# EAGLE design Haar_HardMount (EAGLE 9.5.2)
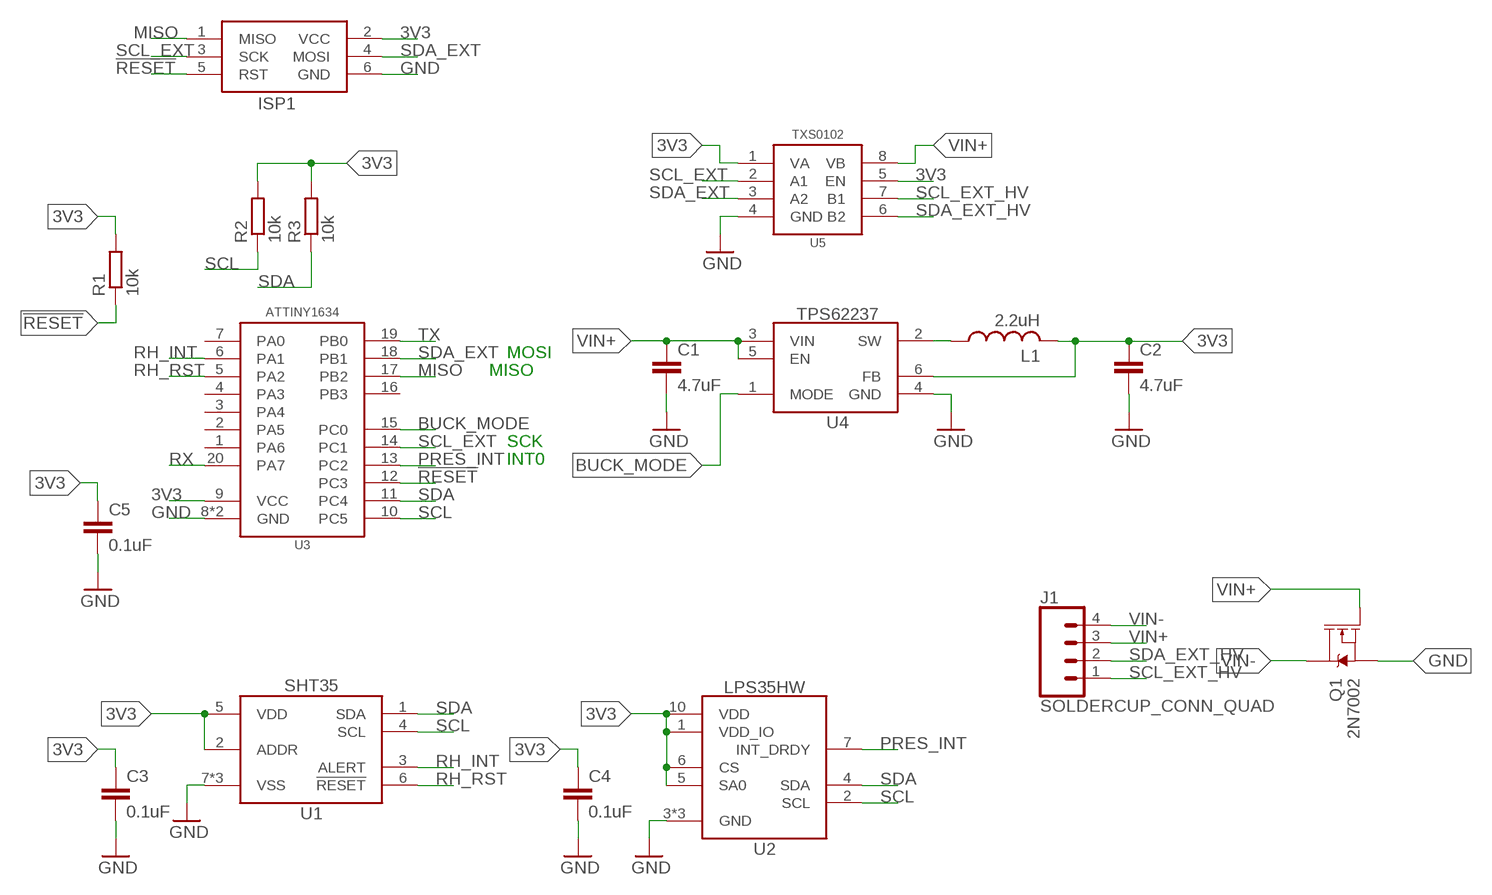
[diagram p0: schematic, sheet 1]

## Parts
C1  4.7uF  C-EUC0402  [C0402]
C2  4.7uF  C-EUC0402  [C0402]
C3  0.1uF  C-EU0.1UFC0402  [C0402]
C4  0.1uF  C-EU0.1UFC0402  [C0402]
C5  0.1uF  C-EU0.1UFC0402  [C0402]
ISP1  AVRISP1.27MM  [2X3_1.27]
J1  SOLDERCUP_CONN_QUAD  [SOLDERCUP_CONN_QUAD]
L1  2.2uH  INDUCTOR0805  [0805]
Q1  2N7002  MOSFET-NCH-2N7002PW  [SOT323]
R1  10k  R-EU_10KR0402  [R0402]
R2  10k  R-EU_10KR0402  [R0402]
R3  10k  R-EU_10KR0402  [R0402]
U1  SHT35DFN  [DFN_8_2.5X2.5]
U2  LPS35HW  [CCLGA10L]
U3  ATTINY1634QFN  [QFN20]
U4  TPS62237DRY  [DRY0006A]
U5  TXS0102DQM  [DQM_R-PX2SON-N8]

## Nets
3V3: C2.1 C3.1 C4.1 C5.1 ISP1.2(VCC) L1.2 R1.2 R2.2 R3.2 U1.2(ADDR) U1.5(VDD) U2.1(VDD_IO) U2.5(SA0) U2.6(CS) U2.10(VDD) U3.9(VCC) U4.6(FB) U5.1(VA) U5.5(EN)
!RESET: ISP1.5(RST) R1.1 U3.12(PC3)
BUCK_MODE: U3.15(PC0) U4.1(MODE)
GND: C1.2 C2.2 C3.2 C4.2 C5.2 ISP1.6(GND) Q1.2(S) U1.7(VSS) U1.8(VSS) U1.EP(VSS) U2.3(GND) U2.8(GND) U2.9(GND) U3.8(GND) U3.EP(GND) U4.4(GND) U5.4(GND)
MISO: ISP1.1(MISO) U3.17(PB2)
N$1: L1.1 U4.2(SW)
PRES_INT: U2.7(INT_DRDY) U3.13(PC2)
RH_INT: U1.3(ALERT) U3.6(PA1)
RH_RST: U1.6(!RESET) U3.5(PA2)
RX: U3.20(PA7)
SCL: R2.1 U1.4(SCL) U2.2(SCL) U3.10(PC5)
SCL_EXT: ISP1.3(SCK) U3.14(PC1) U5.2(A1)
SCL_EXT_HV: J1.1 U5.7(B1)
SDA: R3.1 U1.1(SDA) U2.4(SDA) U3.11(PC4)
SDA_EXT: ISP1.4(MOSI) U3.18(PB1) U5.3(A2)
SDA_EXT_HV: J1.2 U5.6(B2)
TX: U3.19(PB0)
VIN+: C1.1 J1.3 Q1.1(G) U4.3(VIN) U4.5(EN) U5.8(VB)
VIN-: J1.4 Q1.3(D)
Unconnected: U3.1(PA6) U3.2(PA5) U3.3(PA4) U3.4(PA3) U3.7(PA0) U3.16(PB3)

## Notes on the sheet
- MOSI
- MISO
- SCK
- INT0

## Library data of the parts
C1 C2 = bschulz_passives:C-EU: CAPACITOR, European symbol; DIGIKEY: 490-14306-1-ND; MF: Murata; MPN: GRM155R61A475MEAAD
C3-C5 = bschulz_passives:C-EU: CAPACITOR, European symbol; DIGIKEY: 490-4759-1-ND; MF: Murata; MPN: GCM155R71C104KA55D
ISP1 = bschulz:AVRISP: AVR ISP HEADER Standard 6 pin header for AVR programming
J1 = bschulz:SOLDERCUP_CONN_QUAD
L1 = bschulz:INDUCTOR: Genaric inductor; DIGIKEY: 732-2953-1-ND; MF: Wurth; MPN: 74479775222
Q1 = bschulz:MOSFET-NCH: N-channel MOSFETs Voltage controlled devices that allow control of high current outputs. SparkFun Products: SparkFun OpenScale SparkFun Digital Sandbox SparkFun Monster Moto Shield SparkFun MOSFET Power Controller; DIGIKEY: 2N7002W-FDICT-ND; MF: Diodes Incorporated; MPN: 2N7002W-7-F; PROD_ID: TRANS-11151
R1-R3 = bschulz_passives:R-EU_: RESISTOR, European symbol; DIGIKEY: 311-10.0KHRCT-ND; MF: Yageo; MPN: RC0603FR-0710KL; VALUE_PART: 10k
U1 = bschulz:SHT3*: SHT3x - Digital Humidity and Temperature Sensor Characteristics (for SHT35): Vcc: 2.15V ~ 5.5V Humidity Resolution: 0.01% RH Humidity Accuracy: &plusmn;1.5% RH Temperature Resolution: 0.01°C Temperature Accuracy: 0.1°C Operating Temperature: -40°C to 125°C Digikey: 1649-1065-1-ND (SHT30)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; DIGIKEY: 1649-1067-1-ND; DISP: SHT35; MF: Sensirion; MPN: SHT35-DIS-F2.5KS
U2 = bschulz:LPS3*HW: LPS3xHW - Digital Water Resistant Pressure Sensor Characteristics: Vcc: 1.7V ~ 3.6V Pressure Range: 260 ~ 1260 mBar Pressure Resolution: 0.24 &mu;Bar Pressure Accuracy: relative &plusmn;0.1 mBar, abs &plusmn; 1 mBar Temperature Resolution: 0.01°C Temperature Accuracy: 1.5°C Operating Temperature: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; DIGIKEY: 497-16706-1-ND; DISP: LPS35HW; MF: ST; MPN: LPS35HWTR
U3 = bschulz:ATTINY1634: ATtiny1634 8 bit AVR Microcontroller Features: Vcc: 1.8 ~ 5.5V Clock: Up to 16MHz, Internal 8MHz FRC, 32kHz RC Flash Memory: 16K SRAM: 1K EEPROM: 256B ADC: 10b, 12 port USART: Yes, x2 SPI: Yes I2C: Yes, slave only Notes: 2 analog comp. Digikey: ATTINY1634R-MURCT-ND (QFN) ATTINY1634R-SU-ND (SOIC); DIGIKEY: ATTINY1634-MURCT-ND; MF: Atmel; MPN: ATTINY1634-MUR
U4 = bschulz:TPS6223*: TPS6223xx - Ultra Small Step Down Converter (Buck) Characteristics: Vin: 2.05V ~ 6V Vout: 1V ~ 3.3V (fixed increments) IQ: 22&mu;A Output Current: 500 mA Operating Temperature: -40°C to 85°C Digikey: TPS62237 (3.3V Fixed); DIGIKEY: 296-39454-1-ND; DISP: TPS62237; MF: TI; MPN: TPS62237DRYR
U5 = bschulz:TXS0102: TXS0102 - 2 Channel Bidirectional Voltage Level Translator Characteristics: Vcc: 1.65 ~ 3.6V (Port A), 2.3 ~ 5.5V (Port B) IQ: 14.4&mu;A Output Current: 50mA Output Type: Open Drain/Push-Pull Operating Temperature: -40°C to 85°C Digikey: 296-28368-1-ND (DQE) 296-28435-1-ND (DQM) 296-21931-1-ND (DCU); DIGIKEY: 296-28435-1-ND; MF: TI; MPN: TXS0102DQMR

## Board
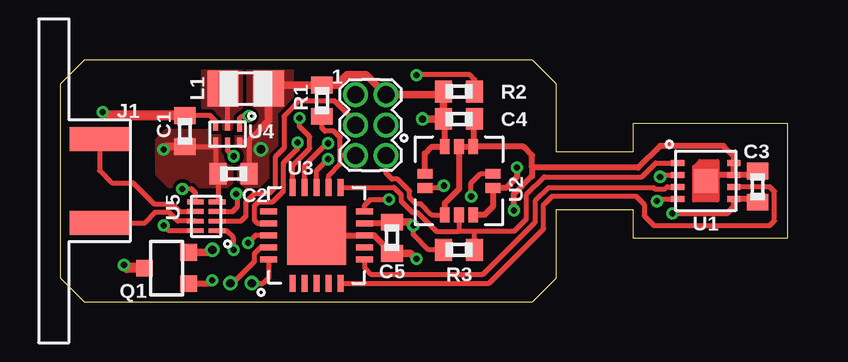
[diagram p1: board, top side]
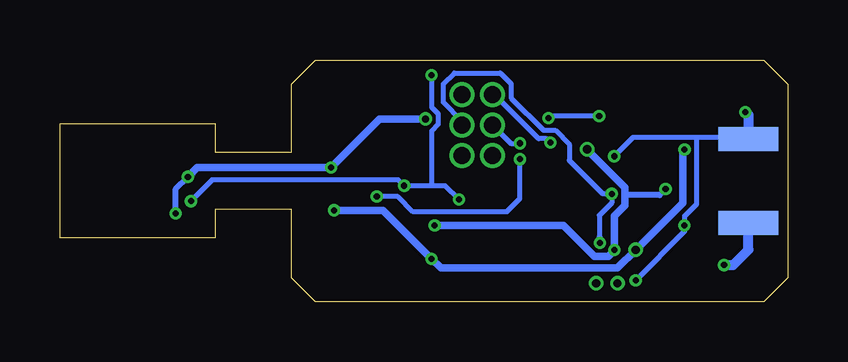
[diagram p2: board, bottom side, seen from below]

Size 30.35 x 10.08 mm. Coordinates in mm from the lower left corner, seen from the top.
Outline: 20.7,6.23 20.7,9.08 19.7,10.08 1,10.08 0,9.08 0,1 1,0 19.7,0 20.7,1 20.7,3.85 23.88,3.85 23.88,2.66 30.35,2.66 30.35,7.42 23.88,7.42 23.88,6.23 20.7,6.23
Copper layers (1*16): Top 0.035559375mm / dielectric 1.6mm / Bottom 0.035559375mm
Design rules "oshpark-2layer": minimum track width 6mil, minimum drill 10mil, track to track 6mil, track to pad 6mil, pad to pad 6mil, via to via 6mil, smd to smd 6mil, copper to edge 15mil, drill to drill 6mil, minimum pad ring 5mil, minimum via ring 5mil, stop-mask expansion 2.5mil, vias tented up to drill 0mil, thermal gap 10mil

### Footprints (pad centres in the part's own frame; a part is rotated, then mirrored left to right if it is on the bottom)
C0402 = smd 0.7 x 0.9: 1 -0.65,0; 2 0.65,0
2X3_1.27 = drill 0.7 pad 1.05: 1 -1.27,-0.635; 2 -1.27,0.635; 3 0,-0.635; 4 0,0.635; 5 1.27,-0.635; 6 1.27,0.635
SOLDERCUP_CONN_QUAD = smd 1 x 2.5: 1 1.75,1.27; 2 -1.75,1.27 | smd 1 x 2.5 bottom: 3 -1.75,1.27; 4 1.75,1.27
0805 = smd 1.3 x 1.5: 1 -0.95,0; 2 0.95,0
SOT323 = smd 0.7 x 0.7: 1 -0.65,-0.925; 2 0.65,-0.925; 3 0,0.925
R0402 = smd 0.7 x 0.9: 1 -0.65,0; 2 0.65,0
DFN_8_2.5X2.5 = smd 0.55 x 0.25: 1 -1.175,0.75; 2 -1.175,0.25; 3 -1.175,-0.25; 4 -1.175,-0.75; 5 1.175,-0.75; 6 1.175,-0.25; 7 1.175,0.25; 8 1.175,0.75 | smd 1 x 1: EP 0,0
CCLGA10L = smd 0.63 x 0.4: 1 -1.42,0.3; 2 -1.42,-0.3; 6 1.42,-0.3; 7 1.42,0.3 | smd 0.4 x 0.63: 3 -0.6,-1.42; 4 0,-1.42; 5 0.6,-1.42; 8 0.6,1.42; 9 0,1.42; 10 -0.6,1.42
QFN20 = smd 0.7 x 0.25: 1 -2.032,0.968; 2 -2.032,0.468; 3 -2.032,-0.032; 4 -2.032,-0.532; 5 -2.032,-1.032; 11 1.968,-1.032; 12 1.968,-0.532; 13 1.968,-0.032; 14 1.968,0.468; 15 1.968,0.968 | smd 0.25 x 0.7: 6 -1.032,-2.032; 7 -0.532,-2.032; 8 -0.032,-2.032; 9 0.468,-2.032; 10 0.968,-2.032; 16 0.968,1.968; 17 0.468,1.968; 18 -0.032,1.968; 19 -0.532,1.968; 20 -1.032,1.968 | smd 2.45 x 2.45: EP -0.032,-0.032
DRY0006A = smd 0.35 x 0.2: 1 -0.275,0.5 | smd 0.3 x 0.2: 2 -0.3,0; 3 -0.3,-0.5; 4 0.3,-0.5; 5 0.3,0; 6 0.3,0.5
DQM_R-PX2SON-N8 = smd 0.2 x 0.7: 1 -0.6,-0.45; 2 -0.2,-0.45; 3 0.2,-0.45; 4 0.6,-0.45; 5 0.6,0.45; 6 0.2,0.45; 7 -0.2,0.45; 8 -0.6,0.45

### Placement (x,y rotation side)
C1  5.21,7.11 270 top
C2  7.24,5.33 180 top
C3  29.08,4.8 90 top
C4  16.64,7.62 0 top
C5  13.84,2.67 270 top
ISP1  12.95,7.37 270 top
J1  0.38,5.04 270 top
L1  7.75,8.89 0 top
Q1  4.45,1.4 90 top
R1  10.92,8.38 90 top
R2  16.64,8.76 180 top
R3  16.64,2.16 180 top
U1  26.92,5.04 0 top
U2  16.64,5.04 0 top
U3  10.67,2.79 90 top
U4  6.99,6.99 270 top
U5  6.1,3.56 90 top

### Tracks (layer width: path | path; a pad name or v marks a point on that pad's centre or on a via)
3V3  (via drill 0.25, 0.3, 0.35)
  Top 0.2: U5.5 5.65,4.54 5.48,4.7 v5.1,4.7 | 6.76,2.96 U5.1 6.95,2.96 7.24,2.67 v7.24,2.16 | 8.38,7.24 7.89,6.75 7.89,6.68 | 7.89,6.68 C2.1 | U4.6 7.89,6.68 | v25.02,5.21 25.1,5.29 U1.2 | R3.2 15.37,2.16 14.73,2.79 v14.73,3.17
  Top 0.254: U2.1 15.22,6.19 15.49,6.46 U2.10 16.04,7.57 C4.1 | 28.93,4.25 C3.1 28.94,4.29 U1.5 28.1,3.97 27.81,3.68 v25.53,3.68 | v19.05,5.59 19.05,5.21 18.59,4.74 U2.6 18.06,3.97 17.71,3.62 U2.5 | C5.1 13.79,3.26 U3.9
  Top 0.305: 8.38,7.24 8.7,7.55 L1.2 8.84,9.03 R1.2 11.54,9.03 11.97,9.47 12.76,9.47 ISP1.2 15.86,8.64 R2.2 C4.1 v15.11,7.62 | v14.73,3.17 14.59,3.32 C5.1
  Bottom 0.254: v25.53,3.68 25.53,4.7 v25.02,5.21 | v19.05,5.59 | v5.1,4.7 5.36,4.45 6.79,4.45
  Bottom 0.305: v19.05,5.59 24.64,5.59 v25.02,5.21 | v14.73,3.17 9.35,3.17 8.07,1.89 7.48,1.89 7.24,2.13 v7.24,2.16 7.24,3.56 6.79,4.01 6.79,4.45 6.79,4.76 v8.38,6.35 | v19.05,5.59 17.02,7.62 v15.11,7.62
  pour Top (rank 2, no thermals): 7.87,9.65 7.87,7.24 7.75,7.11 7.37,7.11 7.37,5.21 7.75,4.83 8.26,4.83 9.65,6.22 9.65,9.78 9.53,9.91 8.13,9.91
!RESET
  Top 0.2: ISP1.5 11.68,6.1 | 11.68,6.1 11.68,6.84 11.41,7.11 11.05,7.11 10.92,7.24 R1.1 | 11.68,6.1 11.68,6.09 11.68,5.73 11.2,5.25 U3.12
BUCK_MODE  (via drill 0.25)
  Top 0.2: U4.1 7.49,7.64 7.58,7.74 v7.87,7.74 | v9.98,7.65 9.98,7.31 10.41,6.88 10.41,6.39 9.7,5.68 U3.15
  Bottom 0.2: v7.87,7.74 9.9,7.74 v9.98,7.65
GND  (via drill 0.25, 0.35)
  Top 0.2: ISP1.6 13.59,5.37 13.84,5.11 14.07,5.11 14.58,4.61 14.58,4.34 14.84,4.07 15.05,4.07 15.5,3.62 U2.3 | U4.4 6.49,6.48 | 6.49,6.48 6.49,5.44 C2.2 6.59,4.2 U5.4 | C1.2 6.47,6.46 6.49,6.48
  Top 0.254: U2.8 U2.9 16.64,4.7 16.04,4.1 U2.3 | C4.2 17.24,7.57 U2.8 | U1.7 U1.8 28.1,6.06 27.66,6.5 25.01,6.5 24.1,5.59 19.68,5.59 | 28.94,5.25 C3.2 28.98,5.29 U1.7 | C5.2 13.1,2.76 U3.8 U3.EP | v18.92,3.81 v18.93,3.81 18.93,4.47 19.68,5.24 19.68,5.59 | 19.68,5.59 19.68,6.1 19.32,6.46 U2.8 | 27.17,5.25 U1.EP 27.17,5.29 U1.7
  Top 0.305: v4.32,6.35 4.43,6.46 C1.2 | v14.86,1.78 14.62,2.02 C5.2 | v6.35,2.16 6.24,2.05 Q1.2
  Bottom 0.305: v4.32,6.35 4.39,6.27 4.39,4.12 v6.35,2.16 7.11,1.4 14.48,1.4 v14.86,1.78 16.89,3.81 v18.92,3.81
  pour Top (no thermals): 4.45,7.11 6.6,7.11 6.73,6.99 6.73,6.22 7.11,5.84 7.11,4.95 6.99,4.83 4.57,4.83 4.06,5.33 4.06,6.73
MISO  (via drill 0.25)
  Top 0.2: v9.91,6.64 9.91,6.39 9.32,5.8 9.32,4.62 8.84,4.14 8.24,4.14 8.1,3.99 8.1,3.4 8.24,3.26 U3.17
  Bottom 0.2: ISP1.1 12.24,8.64 10.39,6.79 10.06,6.79 v9.91,6.64
N$1
  Top 0.2: U4.2 6.99,8.7 L1.1
  pour Top (rank 3, no thermals): 6.73,7.37 6.86,7.24 7.11,7.24 7.24,7.37 7.24,7.75 7.62,8.13 7.62,9.65 7.49,9.78 6.1,9.78 5.97,9.65 5.97,8.13 6.22,7.87 6.6,7.87 6.73,7.75
PRES_INT  (via drill 0.25)
  Top 0.2: v17.14,4.38 17.14,4.95 17.53,5.34 U2.7 | U3.13 10.7,5.47 v11.18,5.94
  Bottom 0.2: v17.14,4.38 16.27,4.38 15.63,3.75 11.73,3.75 11.18,4.3 v11.18,5.94
RH_INT
  Top 0.2: U3.6 12.7,1.4 12.95,1.14 17.64,1.14 19.81,3.31 19.81,4.19 20.37,4.75 24.76,4.75 24.81,4.7 25.23,4.7 25.32,4.79 U1.3
RH_RST
  Top 0.2: U3.5 17.89,0.76 20.16,3.04 20.16,4.04 20.53,4.4 24.01,4.4 24.36,4.05 24.36,3.58 24.77,3.17 29.59,3.17 29.79,3.37 29.79,4.6 29.59,4.79 U1.6
RX  (via drill 0.35)
  Top 0.2: U3.20 8.7,1 8.46,0.76 v8,0.76
SCL  (via drill 0.25)
  Top 0.2: U3.10 12.7,4.02 12.94,4.26 v13.72,4.26 | v24.89,4.19 24.99,4.29 U1.4 | v16,4.83 15.91,4.74 U2.2 | v14.86,9.45 14.88,9.46 17.09,9.46 17.29,9.27 R2.1
  Bottom 0.2: v13.72,4.26 14.29,4.83 14.86,4.83 | 14.86,4.83 v16,4.83 16.26,5.09 24,5.09 v24.89,4.19 | v14.86,9.45 14.86,8.12 14.58,7.84 14.58,7.4 14.86,7.12 14.86,4.83
SCL_EXT  (via drill 0.25)
  Top 0.2: ISP1.3 12.32,7.49 11.43,8.38 10,8.38 9.34,7.72 9.34,6.4 8.97,6.04 8.97,4.77 8.69,4.49 8.1,4.49 7.75,4.14 7.75,3.56 7.54,3.36 U5.2 | U3.14 10.2,5.68 11.12,6.6 v11.18,6.6
  Bottom 0.2: ISP1.3 11.56,6.6 v11.18,6.6
SCL_EXT_HV
  Top 0.2: U5.7 4.91,3.36 4.54,3.73 3.98,3.73 3.55,3.29 J1.1
SDA
  Top 0.2: U2.4 16.64,2.93 | 17.29,2.93 18.93,2.93 19.43,3.43 19.43,4.45 20.19,5.21 24.26,5.21 24.84,5.79 U1.1 | 17.29,2.93 16.64,2.93 | U3.11 13.93,4.76 14.22,4.46 14.22,4.32 14.22,4.19 14.69,3.72 14.9,3.72 15.69,2.93 16.64,2.93 | R3.1 17.29,2.93
SDA_EXT  (via drill 0.25)
  Top 0.2: U3.18 8.15,2.76 v7.84,2.45 | 6.61,3.76 U5.3 7.2,3.76 7.39,3.95 7.39,4.46 v7.35,4.5
  Bottom 0.2: ISP1.4 13.59,7.54 14.37,8.31 14.37,9.09 13.91,9.54 12,9.54 11.54,9.09 11.54,8.5 10.19,7.15 9.7,7.15 9.11,6.56 9.11,5.89 7.73,4.5 v7.35,4.5 7.35,4.12 7.87,3.6 7.87,2.71 7.84,2.68 v7.84,2.45
SDA_EXT_HV
  Top 0.2: 5.43,3.76 U5.6 5.01,3.76 4.68,4.08 3.92,4.08 3.05,4.95 2.16,4.95 1.65,5.46 J1.2
TX  (via drill 0.35)
  Top 0.2: U3.19 8.37,2.27 8.1,1.99 8.1,1.66 7.2,0.76 v7.11,0.76
VIN+  (via drill 0.25)
  Top 0.2: U5.8 4.54,2.96 v4.32,3.17 | U4.3 6.49,7.54 6.26,7.76 C1.1 | U4.5 6.99,6.3 7.23,6.06 v7.25,6.06
  Top 0.254: v6.35,0.89 6.21,0.75 Q1.1
  Top 0.406: C1.1 1.93,7.76 v1.78,7.91
  Bottom 0.2: v6.35,0.89 4.32,2.92 v4.32,3.17 4.32,3.56 3.81,4.07 3.81,6.86 | v7.25,6.06 6.45,6.86 3.81,6.86 | J1.3 1.76,6.86 3.81,6.86
  Bottom 0.406: v1.78,7.91 1.65,7.78 J1.3
VIN-  (via drill 0.25)
  Top 0.406: Q1.3 2.79,1.4 v2.67,1.52
  Bottom 0.406: v2.67,1.52 2.29,1.52 1.65,2.16 J1.4

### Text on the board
tDocu: SDA | SCL
bDocu: Vin+ | Project Haar v0.1 / ---------------- / Developed by / Northern Widget and / University of Minnesota | Vin-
